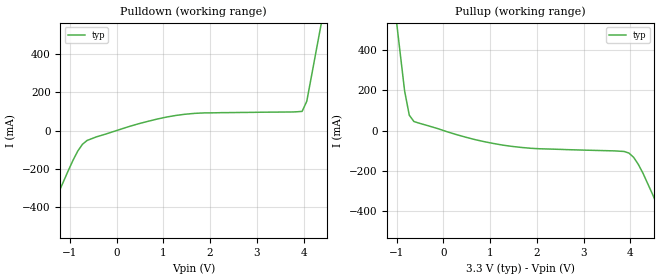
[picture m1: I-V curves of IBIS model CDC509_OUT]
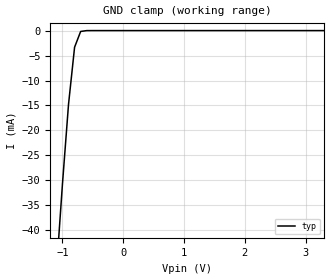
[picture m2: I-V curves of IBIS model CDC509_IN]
[IBIS Ver]   2.1
[File Name]   cdc50901.ibs
[File Rev]   0.1
[Date]   07/16/97
[Source]   File originated at Texas Instruments
[Notes]   The following information corresponds to the
|   CDC509 output buffers and input ESD circuits.
|Revision log: 0.1, 7/16/97 first revision.
[Disclaimer] This information is for modeling purposes only
|and is not guaranteed.
|Property of Texas Instruments Incorporated unauthorized reproduction
|and/or distribution is strictly prohibited.
|This product is protected under copyright law and trade
|secret law as an unpublished work.  Created  1997.
|(C) Copyright 1997 Texas Instruments Incorporated.
|All rights reserved.
|These commodities are under U.S. Government distribution
|license control. As such, they are not to be re-exported
|without prior approval of the U.S. Department of Commerce.
|Please be aware that in the absence of a written agreement
|to the contrary, Texas Instruments ("TI") assumes no
|liability for:  (1) the accuracy of the IBIS Models provided
|to your company;  (2) the proper functioning of these Models
|in your design system or for any resulting applications;
|or (3) infringement of patents, copyrights or intellectual
|property rights resulting from your use of these models.
|TI provides IBIS Models as a service to our customers
|and therefore reserves the right to limit distribution
|of the Models.
|CDC509 IBIS I/O Model
|Mixed Signal Products, Texas Instruments
[Component]   CDC509   | TSSOP - 225mil, PW
[Manufacturer] Texas Instruments
[Package]
|   typ   min   max
R_pkg   0.034   0.031   0.040
L_pkg   2.71n   2.07n   3.51n
C_pkg   0.37p   0.24p   0.48p
[Pin]   signal_name   model_name   R_pin   L_pin   C_pin
 1   AGND   GND   0.035   3.51n   0.48p
 2   VCC   POWER   0.040   3.26n   0.47p
 3   1Y0   CDC509_OUT   0.035   2.96n   0.42p
 4   1Y1   CDC509_OUT   0.031   2.33n   0.32p
 5   1Y2   CDC509_OUT   0.032   2.14n   0.26p
 6   GND   GND   0.031   2.07n   0.24p
 7   GND   GND   0.031   2.07n   0.24p
 8   1Y3   CDC509_OUT   0.032   2.14n   0.26p
 9   1Y4   CDC509_OUT   0.031   2.33n   0.32p
10   VCC   POWER   0.035   2.96n   0.42p
11   1G   CDC509_IN   0.040   3.26n   0.47p
12   FBOUT   CDC509_OUT   0.035   3.51n   0.48p
13   FBIN   CDC509_IN   0.035   3.51n   0.48p
14   2G   CDC509_IN   0.040   3.26n   0.47p
15   VCC   POWER   0.035   2.96n   0.42p
16   2Y3   CDC509_OUT   0.031   2.33n   0.32p
17   2Y2   CDC509_OUT   0.032   2.14n   0.26p
18   GND   GND   0.031   2.07n   0.24p
19   GND   GND   0.031   2.07n   0.24p
20   2Y1   CDC509_OUT   0.032   2.14n   0.26p
21   2Y0   CDC509_OUT   0.031   2.33n   0.32p
22   VCC   POWER   0.035   2.96n   0.42p
23   AVCC   POWER   0.040   3.26n   0.47p
24   CLK   CDC509_IN   0.035   3.51n   0.48p
| Models and submodels in the file (2): CDC509_OUT (Output), CDC509_IN (Input)
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|   Model CDC509_OUT
[Model]   CDC509_OUT
Model_type   Output
Polarity   Non-Inverting
Enable   Active-High
Vmeas = 1.5V
Cref = 30pF
Rref = 500
Vref = 0
|   variable   typ   min   max
C_comp   6.4pF   NA   NA   | typ from real device
[Voltage range]   3.3   NA   NA
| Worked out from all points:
|   slope of the pulldown table from 0 to 0.495 V, typ, clamps not added: 13.4 ohm
|   slope of the pullup table from 0 to 0.495 V, typ, clamps not added: 14.5 ohm
[Pullup]
| Voltage   I(typ)   I(min)   I(max)
-3.3V     5.09A      NA         NA
-1.03V    593mA      NA         NA
-930mV    394mA      NA         NA
-830mV    196mA      NA         NA
-730mV    75.9mA     NA         NA
-630mV    44.6mA     NA         NA
1.27V     -72.4mA    NA         NA
3.87V     -104mA     NA         NA
4.17V     -168mA     NA         NA
4.77V     -475mA     NA         NA
5.27V     -747mA     NA         NA
6.6V      -1.48A     NA         NA
[Pulldown]
|  Voltage   I(typ)   I(min)   I(max)
-3.3V     -1.45A     NA         NA
-2.03V    -763mA     NA         NA
-1.53V    -488mA     NA         NA
-830mV    -107mA     NA         NA
-630mV    -51.6mA    NA         NA
-430mV    -32.9mA    NA         NA
670mV     47.7mA     NA         NA
1.47V     84.8mA     NA         NA
3.97V     99.4mA     NA         NA
4.07V     152mA      NA         NA
4.37V     543mA      NA         NA
6.6V      3.45A      NA         NA
[Ramp]
|  variable   typ   min   max
dV/dt_r   1.60/1.17n   NA   NA   | typ from real device
dV/dt_f   1.60/0.855n   NA   NA   | typ from real device
|   Model CDC509_IN
[Model]   CDC509_IN
Model_type   Input
Polarity   Non-Inverting
Vinl = 0.8V
Vinh = 2.0V
Vmeas = 1.5V
| variable   typ   min   max
C_comp   4.2p   NA   NA   | typ from real device
[Voltage range]   3.3   NA   NA
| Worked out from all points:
|   GND clamp passes 1 mA (typ) near -0.73 V on its own axis
[GND_Clamp]
|  Voltage   I(typ)   I(min)   I(max)
-3.3V     -477mA     NA         NA
-1.1V     -48.3mA    NA         NA
-1V       -30.8mA    NA         NA
-900mV    -14.8mA    NA         NA
-800mV    -3.33mA    NA         NA
-700mV    -173uA     NA         NA
-500mV    -161nA     NA         NA
3.3V      6.3pA      NA         NA
